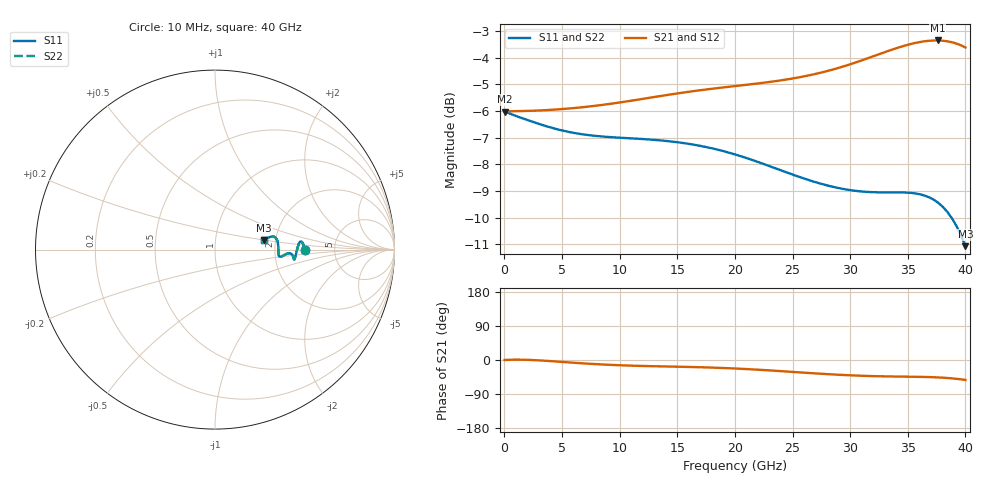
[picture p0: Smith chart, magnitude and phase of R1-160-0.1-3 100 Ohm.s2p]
!version-1
!date-09.2020
# MHz S RI R 50
!Freq ReS11 ImS11 ReS21 ImS21 ReS12 ImS12 ReS22 ImS22
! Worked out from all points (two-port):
!   101 points, 10 MHz to 40 GHz, reference 50 ohm
!   highest |S21| = -3.35 dB at 37.61 GHz (marker M1); lowest = -6.0 dB at 10 MHz (marker M2)
!   |S21| within 3 dB of the highest: start of sweep to end of sweep
!   lowest |S11| = -11.1 dB at 40 GHz (marker M3), VSWR 1.78, Z = 87.1 + j9.98 ohm
!   |S11| at or under -10 dB: 38.79 GHz to end of sweep
!   |S22| runs from -11.1 to -6.0 dB; largest |S21 - S12| = 0
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10  0.4999 0.000489  0.5 0.000158  0.5 0.000158  0.4999 0.000489
410  0.4957 0.0175  0.5004 0.00507  0.5004 0.00507  0.4957 0.0175
1210  0.4872 0.0383  0.5008 0.00783  0.5008 0.00783  0.4872 0.0383
2410  0.4764 0.0453  0.5017 -0.000893  0.5017 -0.000893  0.4764 0.0453
4010  0.4658 0.0289  0.503 -0.026  0.503 -0.026  0.4658 0.0289
6810  0.4526 -0.0191  0.5034 -0.0785  0.5034 -0.0785  0.4526 -0.0191
8410  0.4472 -0.0404  0.5036 -0.1041  0.5036 -0.1041  0.4472 -0.0404
10010  0.4435 -0.0523  0.5049 -0.1245  0.5049 -0.1245  0.4435 -0.0523
11610  0.441 -0.0551  0.5075 -0.14  0.5075 -0.14  0.441 -0.0551
13610  0.4385 -0.0488  0.512 -0.1549  0.512 -0.1549  0.4385 -0.0488
17210  0.4292 -0.0282  0.518 -0.1816  0.518 -0.1816  0.4292 -0.0282
20010  0.4148 -0.0205  0.5157 -0.2133  0.5157 -0.2133  0.4148 -0.0205
22810  0.3955 -0.0254  0.5052 -0.2585  0.5052 -0.2585  0.3955 -0.0254
26810  0.3674 -0.0388  0.4807 -0.337  0.4807 -0.337  0.3674 -0.0388
28810  0.3579 -0.0375  0.4705 -0.3759  0.4705 -0.3759  0.3579 -0.0375
30410  0.3539 -0.0286  0.4666 -0.4043  0.4666 -0.4043  0.3539 -0.0286
32010  0.3527 -0.0117  0.4679 -0.429  0.4679 -0.429  0.3527 -0.0117
33610  0.3524 0.0124  0.4737 -0.4494  0.4737 -0.4494  0.3524 0.0124
36010  0.3457 0.0534  0.4813 -0.4731  0.4813 -0.4731  0.3457 0.0534
37610  0.3298 0.0714  0.4724 -0.4888  0.4724 -0.4888  0.3298 0.0714
38810  0.3077 0.071  0.448 -0.5044  0.448 -0.5044  0.3077 0.071
40000  0.2744 0.0528  0.4002 -0.5242  0.4002 -0.5242  0.2744 0.0528
